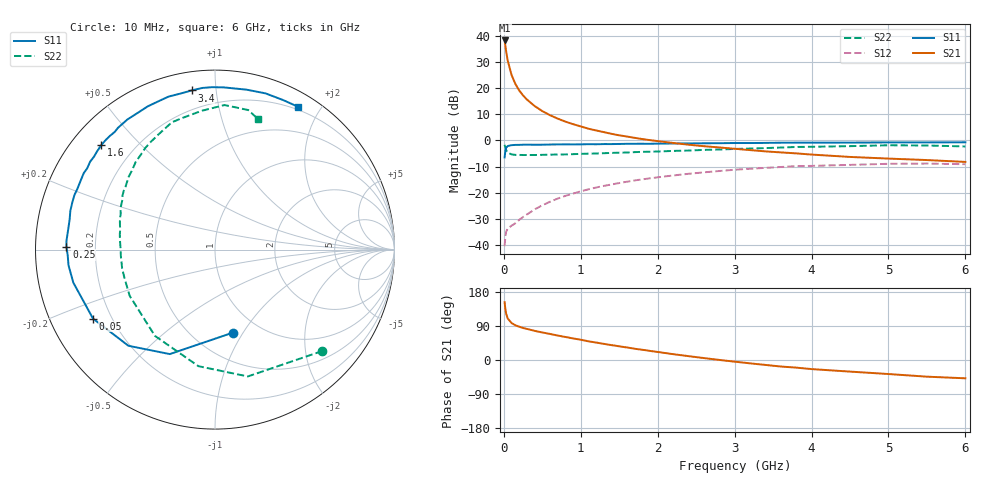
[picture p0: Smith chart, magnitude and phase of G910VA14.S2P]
! SIEMENS Small Signal Semiconductors
! BFG235
! Si NPN RF Bipolar Junction Transistor in SOT223
! VCE = 10 V  IC = 140 mA
! Common Emitter S-Parameters:  July  1994
# GHz  S  MA  R  50
!  f  S11  S21  S12  S22
! GHz  MAG  ANG  MAG  ANG  MAG  ANG  MAG  ANG
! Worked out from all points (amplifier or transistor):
!   40 points, 10 MHz to 6 GHz, reference 50 ohm
!   highest |S21| = 38.2 dB at 10 MHz (marker M1)
!   |S21| within 3 dB of that: start of sweep to 24.59 MHz
!   unconditionally stable (mu >= 1): 452.2 MHz to 1.504 GHz
!   at 200 MHz: K = 0.79, MSG = 24.7 dB, |S12| = -30.4 dB
!   at 1.5 GHz: K = 1.00, MAG = 9.0 dB, |S12| = -16.3 dB
!   at 6 GHz: K = 0.90, MSG = 0.4 dB, |S12| = -9.1 dB
!   S11 on the Smith chart (normalised r, x): 10 MHz: 0.76, -0.91; 50 MHz: 0.13, -0.26; 250 MHz: 0.09, +0.01; 1.6 GHz: 0.09, +0.39; 3.4 GHz: 0.10, +0.86; 6 GHz: 0.17, +1.73
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0.01  0.473 -77.6  81.48 152.7  0.0095 62.8  0.8224 -43.4
0.02  0.6343 -113.4  64.41 133.9  0.0145 50.2  0.73 -75.5
0.03  0.721 -132.0  50.66 122.2  0.0179 41.4  0.656 -98.1
0.05  0.7809 -150.5  33.81 109.6  0.0206 33.8  0.5856 -124.9
0.1  0.8106 -166.9  17.86 97.6  0.0234 35.4  0.5406 -151.6
0.15  0.8208 -173.9  12.01 91.6  0.0261 41.9  0.5286 -162.6
0.2  0.8212 -177.7  8.99 87.8  0.0303 46.5  0.528 -168.6
0.25  0.8277 179.0  7.238 84.5  0.0344 50.6  0.5253 -172.5
0.3  0.829 176.6  6.049 82.0  0.0384 53.5  0.5258 -175.9
0.4  0.8255 172.0  4.544 77.0  0.0479 57.4  0.5257 179.8
0.5  0.8271 168.3  3.634 72.6  0.0575 58.7  0.5294 176.3
0.6  0.8344 165.0  3.032 68.8  0.0671 59.4  0.5336 173.2
0.7  0.8375 161.6  2.61 64.5  0.0772 59.5  0.5376 170.5
0.9  0.8382 156.2  2.045 56.9  0.0963 58.0  0.5459 165.9
1.1  0.8463 149.8  1.675 49.3  0.116 55.5  0.5582 161.3
1.6  0.8602 137.5  1.188 33.1  0.1621 47.5  0.5868 151.3
2.2  0.8739 124.0  0.894 15.4  0.2135 36.9  0.6296 139.7
3.2  0.8903 102.7  0.653 -8.8  0.287 17.6  0.6986 120.8
3.4  0.8961 98.4  0.617 -13.0  0.2984 13.6  0.7134 116.5
4.5  0.9082 78.9  0.483 -30.6  0.3404 -7.4  0.7768 95.5
5.5  0.9155 65.5  0.421 -44.0  0.3609 -25.8  0.7992 76.6
6  0.9206 59.7  0.388 -48.3  0.3505 -32.6  0.7663 71.8
